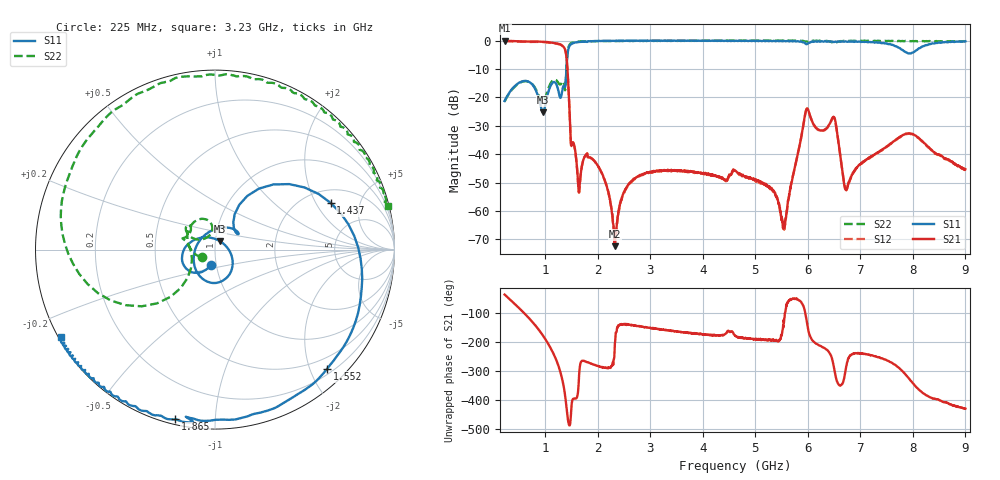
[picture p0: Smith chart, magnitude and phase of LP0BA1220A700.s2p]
!Agilent Technologies,E8358A,US41080443,A.07.50.56
!Agilent E8358A: A.07.50.56
!Date: Tuesday, July 12, 2016 13:38:48
!Correction: S11(Full 2 Port(1,2))
!S21(Full 2 Port(1,2))
!S12(Full 2 Port(1,2))
!S22(Full 2 Port(1,2))
!S2P File: Measurements: S11, S21, S12, S22:
# Hz S  dB  R 50
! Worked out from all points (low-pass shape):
!   1601 points, 225 MHz to 9 GHz, reference 50 ohm
!   highest |S21| = -0.07 dB at 230.5 MHz (marker M1); lowest = -72.4 dB at 2.331 GHz (marker M2)
!   |S21| within 3 dB of the highest: start of sweep to 1.375 GHz
!   lowest |S11| = -25.3 dB at 954.4 MHz (marker M3), VSWR 1.12, Z = 52.7 + j4.92 ohm
!   |S11| at or under -10 dB: start of sweep to 1.402 GHz
!   |S22| runs from -21.8 to 0.0 dB; largest |S21 - S12| = 0.015
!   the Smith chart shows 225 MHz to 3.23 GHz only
!   S11 on the Smith chart (normalised r, x): 225 MHz: 0.94, -0.16; 1.437 GHz: 2.66, +2.68; 1.552 GHz: 0.29, -2.28; 1.865 GHz: 0.02, -0.79; 3.23 GHz: 0.01, -0.26
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2.25e8  -21.29 -105.0  -0.07 -37.3  -0.19 -37.1  -21.49 -149.5
2.304844e8  -21.04 -105.6  -0.07 -38.2  -0.20 -38.0  -21.27 -150.8
6.143906e8  -14.20 -154.3  -0.34 -104.5  -0.45 -104.3  -14.28 127.1
9.544219e8  -25.27 58.7  -0.39 -178.5  -0.52 -178.3  -21.77 126.1
1.223156e9  -15.95 -130.1  -1.03 90.3  -1.15 90.5  -14.23 136.2
1.338328e9  -16.35 49.9  -2.01 16.8  -2.14 17.0  -14.35 161.0
1.437047e9  -3.16 22.0  -15.00 -116.0  -15.12 -116.1  -2.66 -164.9
1.552219e9  -0.80 -46.8  -37.01 -35.6  -37.15 -35.9  -0.54 139.6
1.689328e9  -0.45 -80.8  -44.95 92.3  -44.95 92.9  -0.29 113.9
1.864828e9  -0.25 -103.3  -41.25 85.0  -41.28 85.3  -0.21 91.3
2.331e9  -0.10 -129.2  -72.37 161.9  -69.41 148.8  -0.16 55.9
3.153656e9  -0.09 -149.5  -45.93 -156.0  -45.94 -155.2  -0.06 17.3
3.230438e9  -0.11 -150.5  -45.80 -158.5  -45.83 -158.1  -0.06 14.0
4.6125e9  -0.14 -171.8  -45.72 -179.6  -45.95 -179.3  -0.05 -20.4
5.544844e9  -0.12 166.4  -65.06 -133.0  -66.48 -118.4  -0.10 -32.4
6.076828e9  -0.40 154.0  -28.20 166.8  -28.38 167.7  -0.15 -37.5
6.499125e9  -0.52 138.6  -26.97 69.4  -27.01 69.2  -1.03 -44.1
6.734953e9  -0.37 129.2  -52.05 77.5  -52.67 79.5  -0.13 -44.7
7.541156e9  -1.26 77.1  -36.79 93.4  -36.88 92.9  -0.12 -61.8
7.831828e9  -3.75 3.2  -33.12 52.7  -33.29 53.4  -0.25 -68.4
8.03475e9  -3.81 -98.3  -33.27 9.9  -33.42 10.0  -0.23 -73.7
9e9  -0.27 146.7  -45.28 -70.8  -45.64 -69.5  -0.30 -102.5
